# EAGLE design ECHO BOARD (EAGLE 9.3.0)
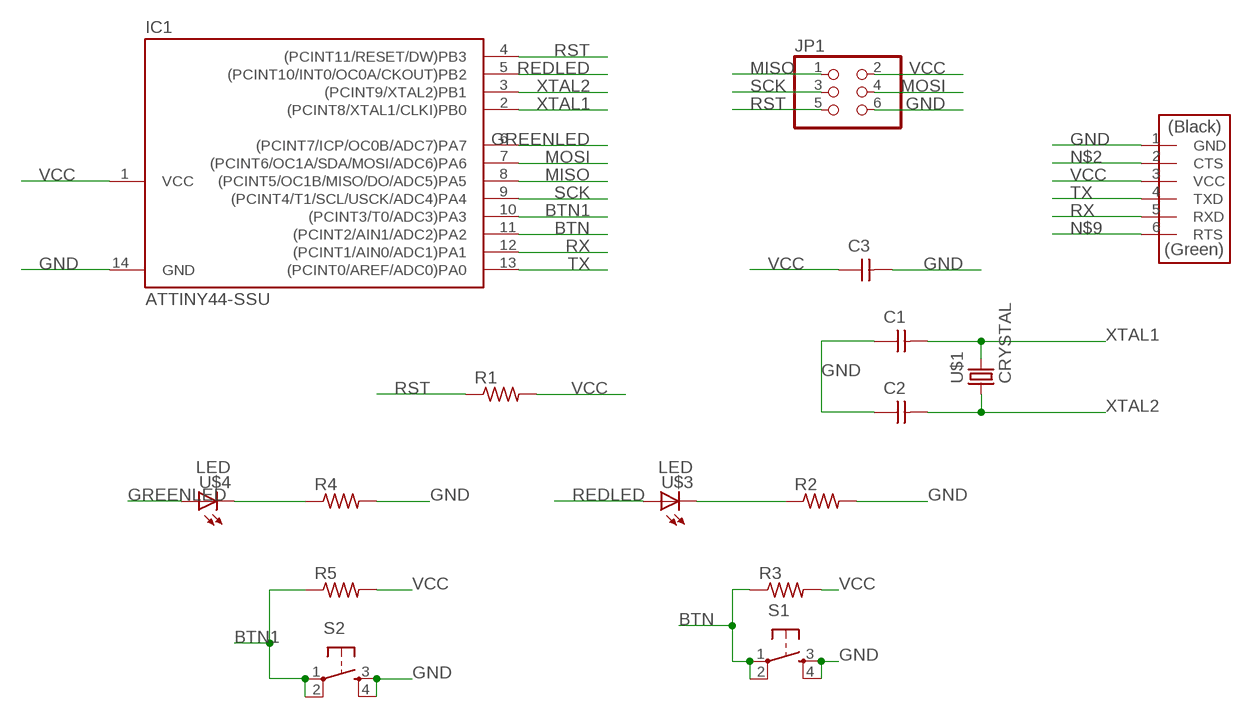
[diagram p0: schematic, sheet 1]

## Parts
C1  CAP-UNPOLARIZEDFAB  [C1206FAB]
C2  CAP-UNPOLARIZEDFAB  [C1206FAB]
C3  CAP-UNPOLARIZEDFAB  [C1206FAB]
IC1  ATTINY44-SSU  [SOIC14]
JP1  PINHD-2X3-SMD  [2X03SMD]
R1  RES-US1206FAB  [R1206FAB]
R2  RES-US1206FAB  [R1206FAB]
R3  RES-US1206FAB  [R1206FAB]
R4  RES-US1206FAB  [R1206FAB]
R5  RES-US1206FAB  [R1206FAB]
S1  6MM_SWITCH6MM_SWITCH  [6MM_SWITCH]
S2  6MM_SWITCH6MM_SWITCH  [6MM_SWITCH]
U$1  CRYSTAL  [2-SMD-5X3MM]
U$2  FTDI-SMD-HEADER  [1X06SMD]
U$3  LED  [LED1206]
U$4  LED  [LED1206]

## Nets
BTN: IC1.11((PCINT2/AIN1/ADC2)PA2) R3.1 S1.1(P) S1.2(P1)
BTN1: IC1.10((PCINT3/T0/ADC3)PA3) R5.1 S2.1(P) S2.2(P1)
GND: C1.1 C2.1 C3.2 IC1.14(GND) JP1.6 R2.2 R4.2 S1.3(S) S1.4(S1) S2.3(S) S2.4(S1) U$2.1(GND)
GREENLED: IC1.6((PCINT7/ICP/OC0B/ADC7)PA7) U$4.1(A)
MISO: IC1.8((PCINT5/OC1B/MISO/DO/ADC5)PA5) JP1.1
MOSI: IC1.7((PCINT6/OC1A/SDA/MOSI/ADC6)PA6) JP1.4
N$1: R2.1 U$3.2(C)
N$2: U$2.2(CTS)
N$4: R4.1 U$4.2(C)
N$9: U$2.6(RTS)
REDLED: IC1.5((PCINT10/INT0/OC0A/CKOUT)PB2) U$3.1(A)
RST: IC1.4((PCINT11/RESET/DW)PB3) JP1.5 R1.1
RX: IC1.12((PCINT1/AIN0/ADC1)PA1) U$2.5(RXD)
SCK: IC1.9((PCINT4/T1/SCL/USCK/ADC4)PA4) JP1.3
TX: IC1.13((PCINT0/AREF/ADC0)PA0) U$2.4(TXD)
VCC: C3.1 IC1.1(VCC) JP1.2 R1.2 R3.2 R5.2 U$2.3(VCC)
XTAL1: C1.2 IC1.2((PCINT8/XTAL1/CLKI)PB0) U$1.P$2
XTAL2: C2.2 IC1.3((PCINT9/XTAL2)PB1) U$1.P$1

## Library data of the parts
C1-C3 = fab:CAP-UNPOLARIZED
IC1 = fab:ATTINY44
JP1 = fab:PINHD-2X3-SMD: PIN HEADER
R1-R5 = fab:RES-US: Resistor (US Symbol)
S1 S2 = fab:6MM_SWITCH: OMRON SWITCH
U$1 = fab:CRYSTAL
U$2 = fab:FTDI-SMD-HEADER
U$3 U$4 = fab:LED: LED

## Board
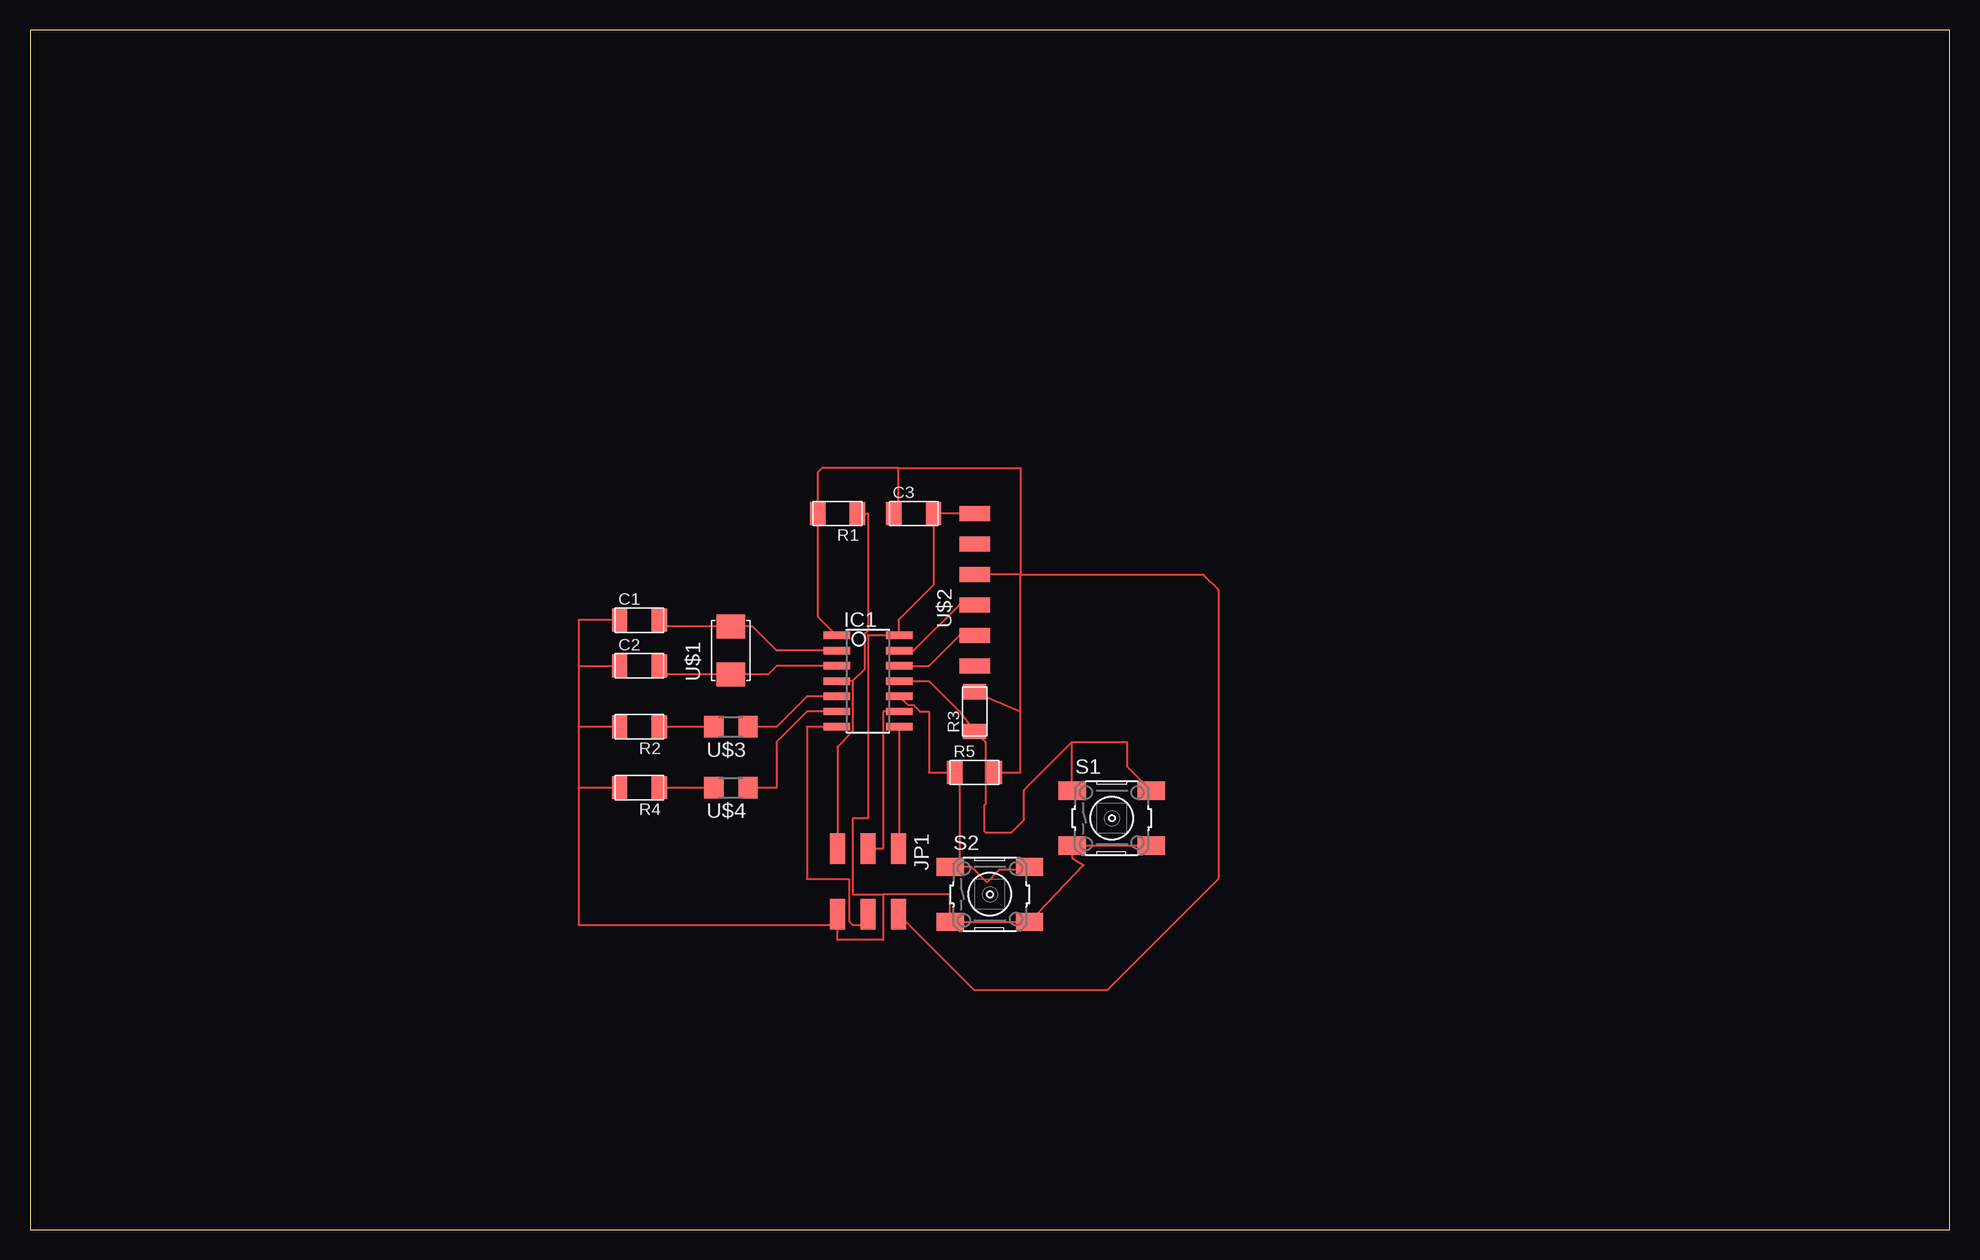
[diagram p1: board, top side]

Size 160 x 100 mm. Coordinates in mm from the lower left corner, seen from the top.
Outline: 0,0 160,0 160,100 0,100 0,0
Copper layers (1*16): Top 0.035mm / dielectric 1.5mm / Bottom 0.035mm
Design rules "default": minimum track width 6mil, minimum drill 0.35mm, track to track 6mil, track to pad 6mil, pad to pad 6mil, via to via 6mil, smd to smd 6mil, copper to edge 40mil, drill to drill 6mil, minimum pad ring 10mil, minimum via ring 8mil, stop-mask expansion 4mil, vias tented up to drill 0mil, thermal gap 10mil

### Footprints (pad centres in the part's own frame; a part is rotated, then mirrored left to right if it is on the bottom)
C1206FAB = smd 1.27 x 1.905: 1 -1.651,0; 2 1.651,0
SOIC14 = smd 0.61 x 2.21: 1 -3.81,-2.603; 2 -2.54,-2.603; 3 -1.27,-2.603; 4 0,-2.603; 5 1.27,-2.603; 6 2.54,-2.603; 7 3.81,-2.603; 8 3.81,2.603; 9 2.54,2.603; 10 1.27,2.603; 11 0,2.603; 12 -1.27,2.603; 13 -2.54,2.603; 14 -3.81,2.603
2X03SMD = smd 2.54 x 1.27: 1 -2.54,2.54; 2 2.92,2.54; 3 -2.54,0; 4 2.92,0; 5 -2.54,-2.54; 6 2.92,-2.54
R1206FAB = smd 1.27 x 1.905: 1 -1.651,0; 2 1.651,0
6MM_SWITCH = smd 2.286 x 1.524: 1 -3.302,2.286; 2 3.302,2.286; 3 -3.302,-2.286; 4 3.302,-2.286
2-SMD-5X3MM = smd 2 x 2.4: P$1 -2,0; P$2 2,0
1X06SMD = smd 2.54 x 1.27: 1 0,6.35; 2 0,3.81; 3 0,1.27; 4 0,-1.27; 5 0,-3.81; 6 0,-6.35
LED1206 = smd 1.6 x 1.803: 1 -1.422,0; 2 1.422,0

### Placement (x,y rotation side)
C1  50.8,50.8 0 top
C2  50.8,46.99 0 top
C3  73.66,59.69 0 top
IC1  69.85,45.72 270 top
JP1  69.85,29.21 270 top
R1  67.31,59.69 180 top
R2  50.8,41.91 180 top
R3  78.74,43.18 90 top
R4  50.8,36.83 180 top
R5  78.74,38.1 0 top
S1  90.17,34.29 0 top
S2  80.01,27.94 0 top
U$1  58.42,48.26 90 top
U$2  78.74,53.34 0 top
U$3  58.42,41.91 180 top
U$4  58.42,36.83 180 top

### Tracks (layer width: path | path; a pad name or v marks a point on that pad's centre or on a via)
BTN
  Top 0.152: IC1.11 74.93,45.72 77.47,43.18 R3.1 79.63,40.64 79.63,35.44 79.53,35.34 79.53,33.24 79.66,33.11 81.8,33.11 82.86,34.16 82.86,36.63 86.87,40.64 | S1.1 86.87,40.64 | 86.87,40.64 91.44,40.64 91.44,38.61 S1.2
BTN1
  Top 0.152: IC1.10 73.19,43.71 73.65,43.71 74.19,43.18 74.93,43.18 74.93,38.1 R5.1 77.47,37.72 77.47,30.99 S2.1 78.49,30.23 79.76,28.96 80.77,29.97 83.06,29.97 S2.2
GND
  Top 0.152: U$2.1 C3.2 75.31,53.72 72.39,50.8 72.39,49.59 IC1.14 69.85,49.53 69.85,34.29 68.58,34.29 68.58,27.94 71.12,27.94 | C1.1 45.72,50.8 45.72,46.99 | 45.72,46.99 C2.1 | 45.72,46.99 45.72,41.91 | 45.72,41.91 45.72,36.83 | 45.72,36.83 45.72,25.4 67.31,25.4 | 67.31,25.4 JP1.6 | R2.2 45.72,41.91 | R4.2 45.72,36.83 | 67.31,25.4 67.31,24.13 71.12,24.13 71.12,27.94 | 71.12,27.94 76.71,27.94 S2.3 S2.4 87.82,30.39 86.87,30.99 S1.3 S1.4
GREENLED
  Top 0.152: IC1.6 64.77,43.18 62.23,40.64 62.23,36.83 U$4.1
MISO
  Top 0.152: IC1.8 72.45,31.81 JP1.1
MOSI
  Top 0.152: IC1.7 64.77,41.91 64.77,29.21 68.28,29.21 68.28,25.7 68.58,25.4 69.85,25.4 JP1.4
N$1
  Top 0.152: U$3.2 R2.1
N$4
  Top 0.152: U$4.2 R4.1
REDLED
  Top 0.152: IC1.5 64.77,44.45 62.23,41.91 U$3.1
RST
  Top 0.152: R1.1 69.85,59.69 69.85,49.96 69.55,49.66 69.55,46.69 68.58,45.72 | 68.58,45.72 IC1.4 | JP1.5 67.31,40.24 68.58,41.51 68.58,45.72
RX
  Top 0.152: U$2.5 77.47,49.53 74.93,46.99 IC1.12
SCK
  Top 0.152: IC1.9 71.12,43.18 71.12,31.75 JP1.3
TX
  Top 0.152: IC1.13 73.66,48.26 77.47,52.07 U$2.4
VCC
  Top 0.152: C3.1 72.39,60.07 72.39,63.5 | 72.39,63.5 82.55,63.5 82.55,54.61 | 82.55,54.61 U$2.3 | 72.39,63.5 66.04,63.5 65.66,63.12 R1.2 65.66,51.12 IC1.1 | 82.55,54.61 97.79,54.61 99.06,53.34 99.06,29.21 89.79,19.94 78.74,19.94 JP1.2 | 82.55,43.18 82.55,38.1 R5.2 | 82.55,43.18 82.55,54.61 | R3.2 82.55,43.18
XTAL1
  Top 0.152: IC1.2 62.23,48.26 60.23,50.26 U$1.P$2 52.99,50.26 C1.2
XTAL2
  Top 0.152: IC1.3 62.23,46.99 61.5,46.26 U$1.P$1 53.18,46.26 C2.2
